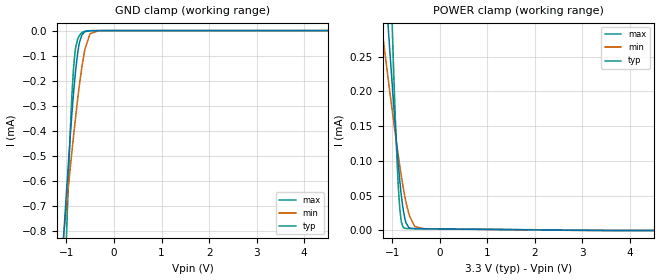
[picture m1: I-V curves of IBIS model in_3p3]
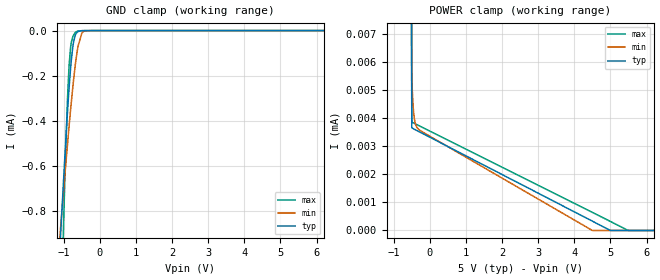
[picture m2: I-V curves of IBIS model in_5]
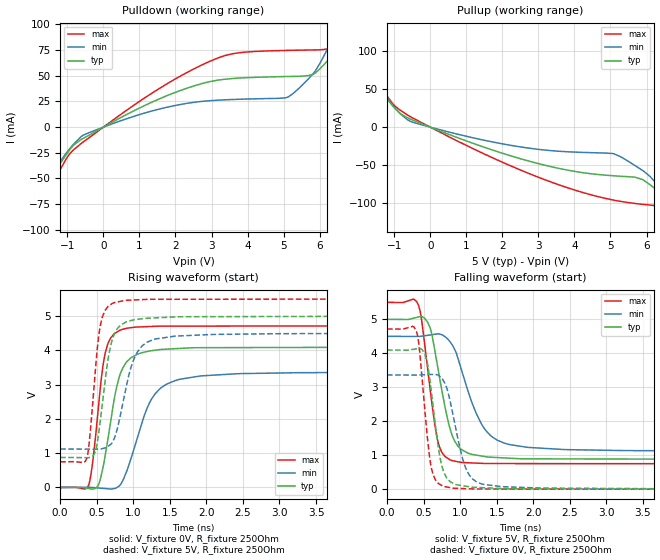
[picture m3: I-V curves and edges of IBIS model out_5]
|Texas Instruments Incorporated
| High-Performance, 8000 VPK Reinforced Quad-Channel Digital Isolator
| Marketing part#   Digital Voltage Range   Package-type   #pins
| ISOW7844FDWE   3.3V-5.5V   SOIC   16
| IS0W7844FDWER   3.3V-5.5V   SOIC   16
| ISOW7844DWE   3.3V-5.5V   SOIC   16
| IS0W7844DWER   3.3V-5.5V   SOIC   16
[IBIS Ver]   4.1
[File name]   isow7844.ibs
[File Rev]   1.0
[Date]   10/19/2016
[Source]
| Texas Instruments Incorporated.
| Analog-eLab Design Center, HPA
| 12500 TI Blvd
| Dallas, TX -75243
[Notes]   Revision History:
| Rev 1.0: 10/19/2016
| - Initial version of the model
| - Model generated from simulations in TISPICE
| - C_comp although listed in numerical order of value are
|   obtained from varying PVT conditions. For PVT conditions for
|   each specific value refer the buffer description under
|   respective [Model]. IBIS model user is responsible for using
|   appropriate C_comp to simulate for Signal Integrity.
|* EXCEPTION:   *
|* - For in_* models there will be leakage current in GROUND clamp  *
|*   because of a resistor(R0) connected to pad.   *
|* - For inf_* models there will be leakage current in POWER clamp   *
|*   because of a resistor(R1) connected to pad.   *
[Disclaimer]
| This model is designed as an aid for customers of Texas Instruments.
| TI and its licensors and suppliers make no warranties, either expressed
| or implied, with respect to this  model, including the warranties of
| merchantability or fitness for a particular purpose. The model is
| provided solely on an "as is" basis. The entire risk as to its quality
| and performance is with the customer.
[Copyright]
(C) Copyright 2016 Texas Instruments Incorporated.All rights reserved.
|   ISOW7844DWE
[Component]   ISOW7844DWE
[Manufacturer]   TI
[Package]   |16 SOIC - DWE package
|   typ   min   max
R_pkg   0.13983   0.12494   0.17928
L_pkg   2.18015nH   1.92454nH   2.85707nH
C_pkg   0.42060pF   0.21450pF   0.61276pF
[Pin]  signal_name   model_name   R_pin   L_pin   C_pin
1   VCC1   POWER   0.09703   2.25823nH  0.63889pF
2   GND1   GND   0.10567   2.15194nH  0.30706pF
3   OUTA   OUT   0.12889   1.99554nH  0.21450pF
4   OUTB   OUT   0.12623   1.94755nH  0.61276pF
5   OUTC   OUT   0.12494   1.92646nH  0.36666pF
6   OUTD   OUT   0.14038   2.18765nH  0.43235pF
7   NC   NC   0.17807   2.83638nH  0.45904pF
8   GND1   GND   0.08216   2.43955nH  0.44498pF
9   GND2   GND   0.10126   2.44074nH  0.40934pF
10   VSEL   NC   0.17928   2.85707nH  0.52717pF
11   IND   IN   0.12883   1.99615nH  0.50841pF
12   INC   IN   0.12617   1.94399nH  0.32633pF
13   INB   IN   0.12498   1.92454nH  0.37783pF
14   INA   IN   0.14050   2.18615nH  0.38097pF
15   GND2   GND   0.08275   2.09014nH  0.75096pF
16   VCC2   POWER   0.09747   2.26909nH  0.67439pF
|   IS0W7844FDWE
[Component]   IS0W7844FDWE
[Manufacturer]   TI
[Package]   |16 SOIC - DWE package
|   typ   min   max
R_pkg   0.2986   0.2007   0.3729
L_pkg   6.1920nH   5.7068nH   6.9814nH
C_pkg   0.3776pF   0.0527pF   0.7658pF
[Pin]  signal_name   model_name   R_pin   L_pin   C_pin
1   VCC1   POWER   0.09703   2.25823nH  0.63889pF
2   GND1   GND   0.10567   2.15194nH  0.30706pF
3   OUTA   OUT   0.12889   1.99554nH  0.21450pF
4   OUTB   OUT   0.12623   1.94755nH  0.61276pF
5   OUTC   OUT   0.12494   1.92646nH  0.36666pF
6   OUTD   OUT   0.14038   2.18765nH  0.43235pF
7   NC   NC   0.17807   2.83638nH  0.45904pF
8   GND1   GND   0.08216   2.43955nH  0.44498pF
9   GND2   GND   0.10126   2.44074nH  0.40934pF
10   VSEL   NC   0.17928   2.85707nH  0.52717pF
11   IND   INF   0.12883   1.99615nH  0.50841pF
12   INC   INF   0.12617   1.94399nH  0.32633pF
13   INB   INF   0.12498   1.92454nH  0.37783pF
14   INA   INF   0.14050   2.18615nH  0.38097pF
15   GND2   GND   0.08275   2.09014nH  0.75096pF
16   VCC2   POWER   0.09747   2.26909nH  0.67439pF
|   Model Selectors
[Model Selector] IN
in_3p3   3.3V digital Input
in_5   5.0V digital Input
[Model Selector] INF
inf_3p3   3.3V digital Input
inf_5   5.0V digital Input
[Model Selector] OUT
out_3p3   3.3V digital 3-state
out_5   5.0V digital 3-state
| Models and submodels in the file (6): in_3p3 (Input), in_5 (Input), inf_3p3 (Input), inf_5 (Input), out_5 (Output), out_3p3 (Output)
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|   in_3p3 Model
[Model]   in_3p3
Model_type   Input
Vinl = 0.99
Vinh = 2.31
|   typ   min   max
|   (nom PVT)   (fast PVT)   (slow PVT)
C_comp   3.281e-15   3.281e-15   3.329e-14
[Model spec]
|subparameter
Vinl   0.99   0.891   1.089
Vinh   2.31   2.079   2.541
| Where nom  PVT is Nominal Process, 3.3V, 27C
|   Fast PVT is Strong Process,  3.63V, -55C
|   Slow PVT is Weak Process,   2.97V, 150C
[Voltage Range]   3.3   2.97   3.63
|Junction Temperature
[Temperature Range]   27   150   -55
[Power Clamp Reference]   3.3   2.97   3.63
[GND Clamp Reference]   0   0   0
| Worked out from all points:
|   GND clamp passes 1 mA (typ) near -1.12 V on its own axis
|   POWER clamp passes 1 mA (typ) near -1.75 V on its own axis
[GND Clamp]
|   Voltage   I(typ)   I(min)   I(max)
-3.3V     -8.284mA   -5.57mA    -16.97mA
-1.076V   -873.6uA   -852.3uA   -1.277mA
-1.002V   -654.2uA   -707.4uA   -840.1uA
-891.3mV  -349uA     -496.6uA   -285.5uA
-853.4mV  -257.3uA   -427.5uA   -158.6uA
-821.7mV  -189.1uA   -371.5uA   -90.58uA
-768.9mV  -98.39uA   -282.7uA   -37.63uA
-719.4mV  -43.62uA   -206.4uA   -17.63uA
-617.1mV  -5.129uA   -80.39uA   -2.416uA
-505.2mV  -641.2nA   -12.81uA   -412.3nA
-330mV    -221.3nA   -470.3nA   -212.8nA
6.6V      0A         0A         0A
[POWER Clamp]
|   Voltage   I(typ)   I(min)   I(max)
-3.3V     2.696mA    1.52mA     6.012mA
-1.242V   453.3uA    304.9uA    851.4uA
-1.198V   407.7uA    280.3uA    746.3uA
-1.049V   257.2uA    198.7uA    400.8uA
-965.9mV  176.8uA    154.6uA    221.3uA
-878.8mV  100.3uA    110.8uA    71.18uA
-842.5mV  72.63uA    93.56uA    33uA
-805.2mV  48.41uA    76.82uA    11.74uA
-737.2mV  18.14uA    49.73uA    3.193uA
-526mV    2.561uA    5.724uA    2.679uA
-330mV    2.416uA    2.488uA    2.553uA
6.6V      0A         0A         0A
|   in_5 Model
[Model]   in_5
Model_type   Input
Vinl = 1.5
Vinh = 3.5
|   typ   min   max
|   (nom PVT)   (fast PVT)   (slow PVT)
C_comp   3.281e-15   3.281e-15   3.455e-14
[Model spec]
|subparameter
Vinl   1.5   1.35   1.65
Vinh   3.5   3.15   3.85
| Where nom  PVT is Nominal Process, 5V, 27C
|   Fast PVT is Strong Process,  5.5V, -55C
|   Slow PVT is Weak Process,   4.5V, 150C
[Voltage Range]   5   4.5   5.5
|Junction Temperature
[Temperature Range]   27   150   -55
[Power Clamp Reference]   5   4.5   5.5
[GND Clamp Reference]   0   0   0
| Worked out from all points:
|   GND clamp passes 1 mA (typ) near -1.12 V on its own axis
[GND Clamp]
|   Voltage   I(typ)   I(min)   I(max)
-5V       -13.99mA   -9.044mA   -29.25mA
-1.112V   -984.3uA   -924.5uA   -1.502mA
-1.062V   -831.8uA   -824.9uA   -1.192mA
-974mV    -572.9uA   -652.8uA   -683.2uA
-908mV    -391.9uA   -527.5uA   -354.9uA
-850mV    -249.6uA   -421.5uA   -149.8uA
-809mV    -164.5uA   -349.6uA   -72.24uA
-740mV    -62.8uA    -237.2uA   -24.38uA
-608mV    -4.229uA   -71.85uA   -2.005uA
-500mV    -598.4nA   -11.5uA    -395.2nA
-347mV    -233.9nA   -591nA     -223.9nA
10V       0A         0A         0A
[POWER Clamp]
|   Voltage   I(typ)   I(min)   I(max)
-5V       185.5mA    66.86mA    305.6mA
-1.007V   217uA      177.2uA    308.5uA
-500mV    3.667uA    5.488uA    3.869uA
-486.5mV  3.656uA    5.003uA    3.86uA
-468.5mV  3.642uA    4.538uA    3.848uA
-428mV    3.613uA    3.98uA     3.822uA
-374mV    3.577uA    3.716uA    3.787uA
-279.5mV  3.514uA    3.578uA    3.726uA
4.5V      333.1nA    0A         645nA
5.005V    0A         0A         319.1nA
5.49V     0A         0A         0A
10V       0A         0A         0A
|   out_5 Model
[Model]   out_5
Model_type   Output
Polarity   Non-Inverting
Vmeas = 2.5
Vref = 5
Cref = 2pF
Rref = 250
|   typ   min   max
C_comp   1.000e-200   NA   NA
|C_comp (ON state)   1.000e-200   NA   NA
|C_comp (OFF state)   1.000e-200   NA   NA
[Voltage Range]   5   4.5   5.5
[Temperature Range]   27   150   -55
[Pullup Reference]   5   4.5   5.5
[Pulldown Reference]   0   0   0
[Power Clamp Reference]   5   4.5   5.5
[GND Clamp Reference]   0   0   0
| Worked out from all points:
|   slope of the pulldown table from 0 to 0.75 V, typ, clamps not added: 52.8 ohm
|   slope of the pullup table from 0 to 0.75 V, typ, clamps not added: 54.8 ohm
|   falling waveform, V_fixture 5V, R_fixture 250Ohm: 20-80 % time 227ps typ, 353ps min, 170ps max; typ from 5 V to 0.878 V
|   rising waveform, V_fixture 0V, R_fixture 250Ohm: 20-80 % time 210ps typ, 342ps min, 147ps max; typ from 0 V to 4.1 V
|   rising waveform, V_fixture 5V, R_fixture 250Ohm: 20-80 % time 161ps typ, 234ps min, 122ps max; typ from 0.878 V to 5 V
|   falling waveform, V_fixture 0V, R_fixture 250Ohm: 20-80 % time 154ps typ, 215ps min, 124ps max; typ from 4.1 V to 0 V
[Pulldown]
|   Voltage   I(typ)   I(min)   I(max)
-5V       -288.8mA   -262.2mA   -333.9mA
-2.54V    -117mA     -112.1mA   -131.5mA
-2.09V    -86.38mA   -85.03mA   -100.4mA
-1.04V    -27.28mA   -25.6mA    -31.38mA
-560mV    -10.96mA   -7.872mA   -14.46mA
3.16V     45.71mA    26.23mA    67.12mA
5.14V     49.34mA    29.7mA     74.77mA
5.845V    51.92mA    53.18mA    75.22mA
6.49V     75.38mA    95.39mA    79.47mA
6.685V    83.25mA    109.4mA    86.48mA
7.165V    106.3mA    144.3mA    108mA
10V       512.8mA    511.9mA    514.1mA
[Pullup]
|   Voltage   I(typ)   I(min)   I(max)
-5V       512.7mA    381.1mA    657.5mA
-3.425V   204.6mA    200mA      221.3mA
-2.12V    100.5mA    104.1mA    104.8mA
-1.04V    27.77mA    28.68mA    30.62mA
-620mV    12.04mA    9.301mA    15.54mA
3.16V     -49.68mA   -29.95mA   -68.57mA
5.26V     -64.33mA   -38.29mA   -97.14mA
5.89V     -68.76mA   -56.77mA   -101.1mA
6.475V    -89.09mA   -85.5mA    -106.4mA
6.685V    -96.8mA    -97.85mA   -114.6mA
7.57V     -131.6mA   -151.1mA   -154.6mA
10V       -299.3mA   -299.6mA   -306.1mA
[Ramp]
R_load = 250
|   typ   min   max
dV/dt_r   2.458/2.09337e-10   2.01688/3.40027e-10   2.83012/1.46155e-10
dV/dt_f   2.47337/2.26564e-10   2.02533/3.51771e-10   2.85107/1.70168e-10
[Falling Waveform]
V_fixture = 5V
V_fixture_min = 4.5V
V_fixture_max = 5.5V
R_fixture = 250Ohm
C_fixture = 0F
|   Time   V(typ)   V(min)   V(max)
0s        5V         4.5V       5.5V
431.1ps   5.071V     4.497V     5.407V
474.5ps   5.084V     4.505V     4.954V
587.1ps   4.764V     4.539V     2.986V
679.1ps   3.77V      4.567V     1.575V
856.1ps   1.826V     4.357V     869.8mV
983.1ps   1.234V     3.759V     801.7mV
1.287ns   978.3mV    1.936V     760.6mV
1.604ns   919.7mV    1.356V     753.5mV
4.9ns     877.7mV    1.124V     748.2mV
[Rising Waveform]
V_fixture = 0V
V_fixture_min = 0V
V_fixture_max = 0V
R_fixture = 250Ohm
C_fixture = 0F
|   Time   V(typ)   V(min)   V(max)
0s        5.119nV    216.1nV    3.276nV
389.6ps   -30.96mV   4.727mV    61.85mV
450.1ps   -48.86mV   -1.736mV   830mV
519.8ps   58.92mV    -14.1mV    2.263V
607.1ps   825.6mV    -29.6mV    3.825V
813.6ps   3.259V     55.84mV    4.586V
967ps     3.784V     833.6mV    4.665V
1.229ns   3.986V     2.502V     4.699V
1.571ns   4.051V     3.118V     4.71V
4.9ns     4.097V     3.361V     4.717V
[Rising Waveform]
V_fixture = 5V
V_fixture_min = 4.5V
V_fixture_max = 5.5V
R_fixture = 250Ohm
C_fixture = 0F
|   Time   V(typ)   V(min)   V(max)
0s        877.7mV    1.123V     748.2mV
364.2ps   870.7mV    1.12V      847.6mV
398.5ps   875mV      1.12V      1.339V
477.8ps   1.034V     1.12V      3.313V
543.8ps   1.865V     1.119V     4.651V
646.7ps   3.625V     1.186V     5.261V
718.1ps   4.341V     1.338V     5.378V
1.004ns   4.89V      3.722V     5.473V
1.272ns   4.948V     4.316V     5.493V
4.9ns     5V         4.498V     5.5V
[Falling Waveform]
|Gnd
V_fixture = 0V
V_fixture_min = 0V
V_fixture_max = 0V
R_fixture = 250Ohm
C_fixture = 0F
|   Time   V(typ)   V(min)   V(max)
0s        4.097V     3.363V     4.717V
401.5ps   4.132V     3.36V      4.647V
441.4ps   4.144V     3.363V     4.146V
513.9ps   3.994V     3.37V      2.407V
596.6ps   3.042V     3.377V     741.1mV
757ps     630.7mV    3.245V     96.2mV
835.6ps   281.6mV    2.84V      57.12mV
1.067ns   89.73mV    673.6mV    15.46mV
1.287ns   45.99mV    160.4mV    4.133mV
4.9ns     19.41uV    1.548mV    -82.18nV
